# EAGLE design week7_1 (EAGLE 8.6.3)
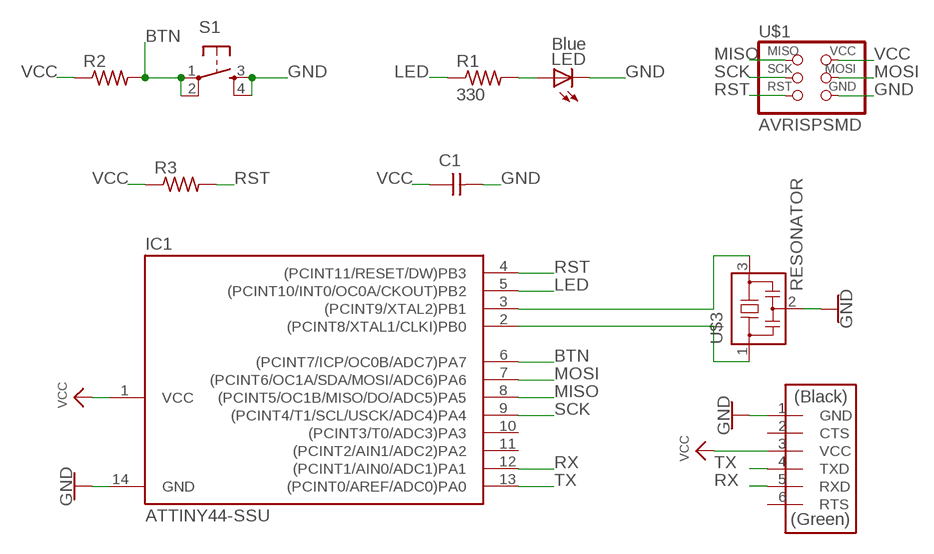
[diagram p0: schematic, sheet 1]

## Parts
C1  CAP-UNPOLARIZEDFAB  [C1206FAB]
IC1  ATTINY44-SSU  [SOIC14]
LED  Blue  LEDFAB1206  [LED1206FAB]
R1  330  RES-US1206FAB  [R1206FAB]
R2  RES-US1206FAB  [R1206FAB]
R3  RES-US1206FAB  [R1206FAB]
S1  6MM_SWITCH6MM_SWITCH  [6MM_SWITCH]
U$1  AVRISPSMD  [2X03SMD]
U$3  RESONATOR  [EFOBM]
U$4  FTDI-SMD-HEADER  [1X06SMD]

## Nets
BTN: IC1.6((PCINT7/ICP/OC0B/ADC7)PA7) R2.2 S1.1(P) S1.2(P1)
GND: C1.2 IC1.14(GND) LED.2(C) S1.3(S) S1.4(S1) U$1.6(GND) U$3.2 U$4.1(GND)
LED: IC1.5((PCINT10/INT0/OC0A/CKOUT)PB2) R1.1
MISO: IC1.8((PCINT5/OC1B/MISO/DO/ADC5)PA5) U$1.1(MISO)
MOSI: IC1.7((PCINT6/OC1A/SDA/MOSI/ADC6)PA6) U$1.4(MOSI)
N$1: IC1.2((PCINT8/XTAL1/CLKI)PB0) U$3.1
N$2: IC1.3((PCINT9/XTAL2)PB1) U$3.3
N$6: LED.1(A) R1.2
RST: IC1.4((PCINT11/RESET/DW)PB3) R3.2 U$1.5(RST)
RX: IC1.12((PCINT1/AIN0/ADC1)PA1) U$4.5(RXD)
SCK: IC1.9((PCINT4/T1/SCL/USCK/ADC4)PA4) U$1.3(SCK)
TX: IC1.13((PCINT0/AREF/ADC0)PA0) U$4.4(TXD)
VCC: C1.1 IC1.1(VCC) R2.1 R3.1 U$1.2(VCC) U$4.3(VCC)
Unconnected: IC1.10((PCINT3/T0/ADC3)PA3) IC1.11((PCINT2/AIN1/ADC2)PA2) U$4.2(CTS) U$4.6(RTS)

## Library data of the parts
C1 = fab:CAP-UNPOLARIZED
IC1 = fab:ATTINY44
LED = fab:LED: LED
R1-R3 = fab:RES-US: Resistor (US Symbol)
S1 = fab:6MM_SWITCH: OMRON SWITCH
U$1 = fab:AVRISP
U$3 = fab:RESONATOR
U$4 = fab:FTDI-SMD-HEADER

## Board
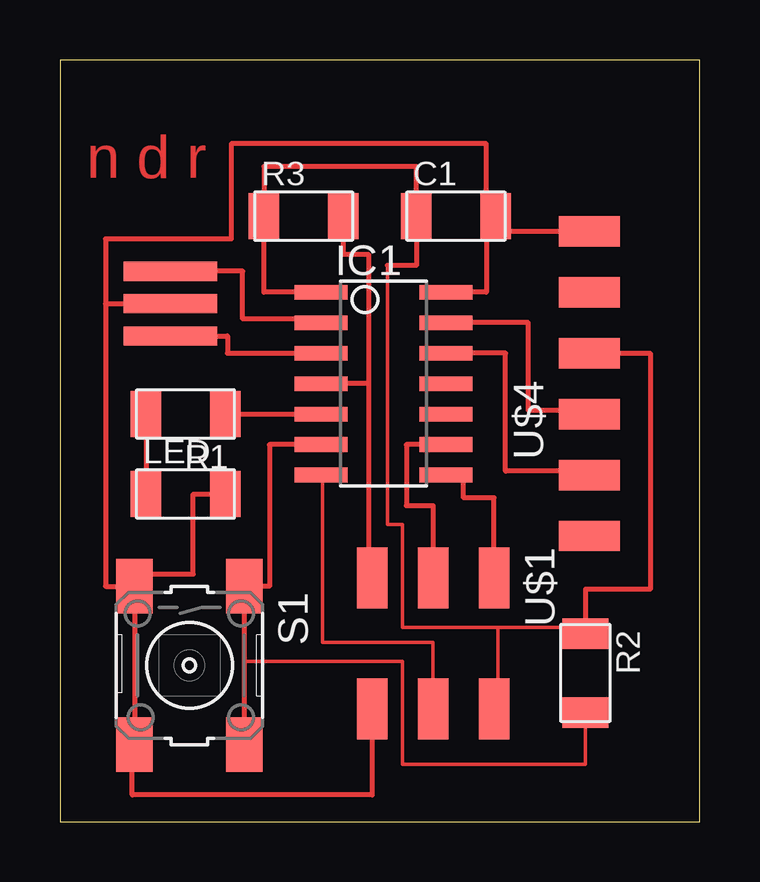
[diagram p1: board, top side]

Size 26.67 x 31.75 mm. Coordinates in mm from the lower left corner, seen from the top.
Outline: 0,0 26.67,0 26.67,31.75 0,31.75 0,0
Copper layers (1*16): Top 0.035mm / dielectric 1.5mm / Bottom 0.035mm
Design rules "default": minimum track width 6mil, minimum drill 0.35mm, track to track 6mil, track to pad 6mil, pad to pad 6mil, via to via 6mil, smd to smd 6mil, copper to edge 40mil, drill to drill 6mil, minimum pad ring 10mil, minimum via ring 8mil, stop-mask expansion 4mil, vias tented up to drill 0mil, thermal gap 10mil

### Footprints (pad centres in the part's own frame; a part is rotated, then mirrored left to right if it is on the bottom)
C1206FAB = smd 1.27 x 1.905: 1 -1.651,0; 2 1.651,0
SOIC14 = smd 0.61 x 2.21: 1 -3.81,-2.603; 2 -2.54,-2.603; 3 -1.27,-2.603; 4 0,-2.603; 5 1.27,-2.603; 6 2.54,-2.603; 7 3.81,-2.603; 8 3.81,2.603; 9 2.54,2.603; 10 1.27,2.603; 11 0,2.603; 12 -1.27,2.603; 13 -2.54,2.603; 14 -3.81,2.603
LED1206FAB = smd 1.27 x 1.905: 1 -1.651,0; 2 1.651,0
R1206FAB = smd 1.27 x 1.905: 1 -1.651,0; 2 1.651,0
6MM_SWITCH = smd 2.286 x 1.524: 1 -3.302,2.286; 2 3.302,2.286; 3 -3.302,-2.286; 4 3.302,-2.286
2X03SMD = smd 2.54 x 1.27: 1 -2.54,2.54; 2 2.92,2.54; 3 -2.54,0; 4 2.92,0; 5 -2.54,-2.54; 6 2.92,-2.54
EFOBM = smd 0.8 x 3.9: 1 -1.35,0; 2 0,0; 3 1.35,0
1X06SMD = smd 2.54 x 1.27: 1 0,6.35; 2 0,3.81; 3 0,1.27; 4 0,-1.27; 5 0,-3.81; 6 0,-6.35

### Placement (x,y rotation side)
C1  16.51,25.24 0 top
IC1  13.49,18.26 270 top
LED  5.24,13.65 0 top
R1  5.24,16.99 180 top
R2  21.91,6.19 270 top
R3  10.16,25.24 0 top
S1  5.4,6.51 270 top
U$1  15.56,7.62 270 top
U$3  4.6,21.59 270 top
U$4  22.07,18.26 0 top

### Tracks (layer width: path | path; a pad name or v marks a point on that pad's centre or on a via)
BTN
  Top 0.152: R2.2 21.91,2.38 14.29,2.38 14.29,6.68 7.68,6.68 7.68,6.67
  Top 0.2: IC1.6 8.73,15.72 8.73,9.81 S1.1 7.68,6.67 S1.2
GND
  Top 0.2: 17.78,25.24 17.78,22.07 IC1.14 | U$4.1 18.16,24.61 C1.2 17.78,25.24 | 6.89,13.97 LED.2 5.56,13.65 5.56,10.32 3.11,10.32 S1.3 | 1.91,21.59 U$3.2 | 1.91,21.59 1.91,24.29 7.14,24.29 7.14,28.26 17.78,28.26 17.78,25.24 | S1.3 S1.4 3.02,3.21 3.02,1.11 13.02,1.11 U$1.6 | 1.91,21.59 1.91,9.81 S1.3
LED
  Top 0.2: R1.1 IC1.5
MISO
  Top 0.2: U$1.1 18.1,13.49 16.83,13.49 16.83,14.45 IC1.8
MOSI
  Top 0.152: IC1.7 10.95,14.45 10.95,7.46 15.56,7.46 U$1.4
N$1
  Top 0.2: IC1.2 10.89,20.95 7.62,20.95 7.62,22.94 U$3.1
N$2
  Top 0.2: IC1.3 6.99,19.53 6.99,20.24 U$3.3
N$6
  Top 0.2: R1.2 LED.1
RST
  Top 0.2: R3.2 11.81,23.65 12.86,23.65 12.86,18.26 | 12.86,18.26 IC1.4 | 12.86,18.26 12.86,10.16 U$1.5
RX
  Top 0.2: U$4.5 22.07,14.61 18.57,14.61 18.57,19.53 IC1.12
SCK
  Top 0.2: IC1.9 14.45,15.72 14.45,13.18 15.56,13.18 U$1.3
TX
  Top 0.2: U$4.4 22.07,17.14 19.53,17.14 19.53,20.8 IC1.13
VCC
  Top 0.152: 13.65,23.18 13.65,12.38 14.29,12.38 14.29,8.1 18.26,8.1 | 18.26,8.1 18.26,4.7 | 18.26,8.1 21.91,8.1 21.91,7.94
  Top 0.2: IC1.1 8.51,22.07 R3.1 8.51,27.3 14.86,27.3 C1.1 14.86,23.18 13.65,23.18 | U$4.3 24.61,19.53 24.61,9.68 21.91,9.68 21.91,7.94 R2.1 | U$1.2 18.26,4.7 18.41,4.7

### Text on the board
Top: n d r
